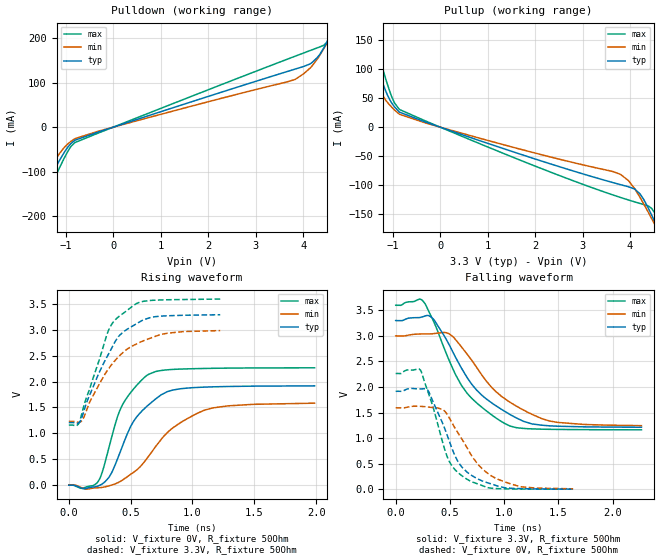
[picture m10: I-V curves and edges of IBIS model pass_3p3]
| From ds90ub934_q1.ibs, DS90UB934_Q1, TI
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|   pass_3p3 Model
[Model]   pass_3p3
Model_type   Output
Polarity   Non-Inverting
Vmeas = 1.65
Vref = 0
Cref = 2pF
Rref = 55
|   typ   min   max
|   (nom PVT)   (fast PVT)   (slow PVT)
C_comp   2.029e-13   1.837e-13   2.456e-13
| Where nom  PVT is Nominal Process, 3.3V, 27C
|   Fast PVT is Strong Process,  3.6V, -40C
|   Slow PVT is Weak Process,   3V, 125C
[Voltage Range]   3.3   3   3.6
|Junction Temperature
[Temperature Range]   27   125   -40
[Pullup Reference]   3.3   3   3.6
[Pulldown Reference]   0   0   0
[Power Clamp Reference]   3.3   3   3.6
[GND Clamp Reference]   0   0   0
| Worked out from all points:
|   slope of the pulldown table from 0 to 0.495 V, typ, clamps not added: 28.8 ohm
|   slope of the pullup table from 0 to 0.495 V, typ, clamps not added: 35.6 ohm
|   falling waveform, V_fixture 3.3V, R_fixture 50Ohm: 20-80 % time 447ps typ, 482ps min, 385ps max; typ from 3.3 V to 1.21 V
|   rising waveform, V_fixture 0V, R_fixture 50Ohm: 20-80 % time 264ps typ, 384ps min, 214ps max; typ from 0 V to 1.92 V
|   rising waveform, V_fixture 3.3V, R_fixture 50Ohm: 20-80 % time 255ps typ, 311ps min, 211ps max; typ from 1.21 V to 3.29 V
|   falling waveform, V_fixture 0V, R_fixture 50Ohm: 20-80 % time 251ps typ, 314ps min, 207ps max; typ from 1.92 V to 0.002 V
[Pulldown]
|   Voltage   I(typ)   I(min)   I(max)
-3.3V     -515.5mA   -439.5mA   -591.7mA
-1.734V   -193.6mA   -159.2mA   -228.7mA
-1.129V   -73.18mA   -58mA      -89.41mA
-920.7mV  -39.61mA   -34.05mA   -47.24mA
-816mV    -29.91mA   -26.38mA   -35.06mA
3.831V    130.6mA    107.3mA    159.5mA
4.148V    142.3mA    132.9mA    172.3mA
4.306V    157.5mA    154.5mA    178.7mA
4.526V    197.6mA    193.2mA    192.8mA
4.613V    217.6mA    209.4mA    207.5mA
4.706V    239.6mA    226.9mA    229.6mA
6.6V      700.6mA    601.5mA    771mA
[Pullup]
|   Voltage   I(typ)   I(min)   I(max)
-3.3V     599.3mA    479.6mA    717mA
-1.911V   244.2mA    185.3mA    301.9mA
-1.674V   185mA      137.1mA    232.1mA
-1.521V   147.3mA    106.9mA    187.4mA
-1.383V   114mA      81.01mA    147.5mA
-1.119V   56.12mA    43.07mA    74.77mA
-861.3mV  25.87mA    22.21mA    30.45mA
3.798V    -99.15mA   -81.35mA   -121.2mA
4.211V    -115.2mA   -121.2mA   -131.6mA
4.527V    -164.1mA   -168.7mA   -149mA
4.772V    -208.2mA   -206.9mA   -194.8mA
6.6V      -545.1mA   -513mA     -568.5mA
[Ramp]
R_load = 50
|   typ   min   max
dV/dt_r   1.15085/2.64025e-10   0.955772/3.8958e-10   1.35908/2.13712e-10
dV/dt_f   1.25533/4.49718e-10   1.0614/4.89618e-10   1.46413/3.85624e-10
[Falling Waveform]
V_fixture = 3.3V
V_fixture_min = 3V
V_fixture_max = 3.6V
R_fixture = 50Ohm
|   Time   V(typ)   V(min)   V(max)
0s        3.3V       3V         3.6V
252.4ps   3.377V     3.039V     3.68V
354.1ps   3.312V     3.046V     3.26V
485.5ps   2.856V     3.048V     2.558V
606.7ps   2.368V     2.784V     2.031V
746.5ps   1.938V     2.383V     1.689V
1.007ns   1.522V     1.77V      1.284V
1.177ns   1.329V     1.55V      1.19V
1.417ns   1.241V     1.335V     1.172V
2.265ns   1.213V     1.244V     1.162V
[Rising Waveform]
V_fixture = 0V
V_fixture_min = 0V
V_fixture_max = 0V
R_fixture = 50Ohm
|   Time   V(typ)   V(min)   V(max)
0s        847.4nV    3.935uV    406.2nV
98.16ps   -53.88mV   -45.46mV   -63.04mV
235.6ps   -18.04mV   -51.37mV   63.01mV
324.4ps   148.8mV    -14.79mV   724.7mV
429.4ps   726.3mV    89.91mV    1.531V
522.9ps   1.23V      245.1mV    1.855V
646ps     1.553V     560.1mV    2.141V
831.9ps   1.83V      1.089V     2.233V
1.096ns   1.893V     1.447V     2.253V
1.987ns   1.917V     1.583V     2.265V
[Rising Waveform]
V_fixture = 3.3V
V_fixture_min = 3V
V_fixture_max = 3.6V
R_fixture = 50Ohm
|   Time   V(typ)   V(min)   V(max)
0s        1.208V     1.231V     1.16V
85.97ps   1.215V     1.212V     1.218V
113.2ps   1.363V     1.268V     1.455V
239.7ps   2.144V     1.92V      2.373V
318.7ps   2.52V      2.238V     2.976V
391.7ps   2.837V     2.454V     3.231V
548.5ps   3.119V     2.728V     3.508V
665.2ps   3.241V     2.844V     3.567V
797.1ps   3.271V     2.934V     3.58V
1.224ns   3.291V     2.985V     3.593V
[Falling Waveform]
V_fixture = 0V
V_fixture_min = 0V
V_fixture_max = 0V
R_fixture = 50Ohm
|   Time   V(typ)   V(min)   V(max)
0s        1.917V     1.593V     2.265V
228.4ps   1.962V     1.622V     2.332V
304.3ps   1.909V     1.607V     1.863V
473.5ps   1.063V     1.469V     641.2mV
572.3ps   545.7mV    1.108V     328.8mV
655.2ps   340mV      819.8mV    197.5mV
797.1ps   161.8mV    401.4mV    71.71mV
955.5ps   53.25mV    182.8mV    10.12mV
1.159ns   11.22mV    46.88mV    3.31mV
1.635ns   1.885mV    7.826mV    1.047mV
